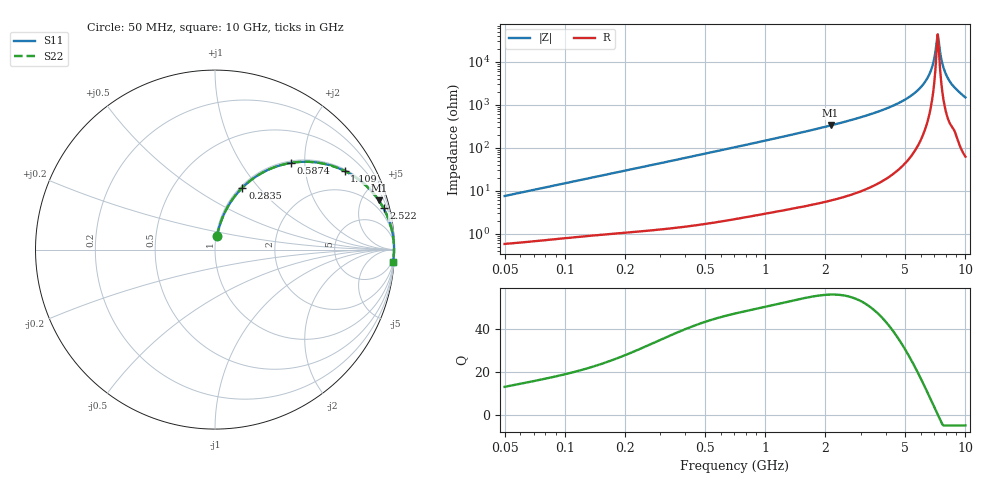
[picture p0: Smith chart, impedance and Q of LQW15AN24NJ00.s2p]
!Murata Part Number: LQW15AN24NJ00
!These Parameters are Measured in Series Mode Connection
!  o--[Z]--o
!Port1  Port2
!  o-------o
!Freq. Start=50[MHz] Stop=10[GHz], 401[Steps]
# Hz S RI R 50
!Freq.(Hz)	S 11(Real)	S 11(Imag)	S 21(Real)	S 21(Imag)	S 12(Real)	S 12(Imag)	S 22(Real)	S 22(Imag)
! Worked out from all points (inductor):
!   401 points, 50 MHz to 10 GHz, reference 50 ohm
!   read as one part in series: L = 23.7 nH near 51.34 MHz
!   highest Q = 56.1 at 2.123 GHz (marker M1), where L = 24.7 nH
!   self-resonance near 7.277 GHz
!   S11 on the Smith chart (normalised r, x): 50 MHz: 1.01, +0.15; 283.5 MHz: 1.02, +0.82; 587.4 MHz: 1.04, +1.71; 1.109 GHz: 1.06, +3.25; 2.522 GHz: 1.15, +8.13; 10 GHz: 2, -30
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5e7  0.0112 0.0737  0.9888 -0.0737  0.9888 -0.0737  0.0112 0.0737
1.214486e8  0.0387 0.1705  0.9613 -0.1705  0.9613 -0.1705  0.0387 0.1705
2.835028e8  0.1527 0.3453  0.8473 -0.3453  0.8473 -0.3453  0.1527 0.3453
2.949953e8  0.1626 0.3549  0.8374 -0.3549  0.8374 -0.3549  0.1626 0.3549
5.874203e8  0.423 0.4831  0.577 -0.4831  0.577 -0.4831  0.423 0.4831
7.071068e8  0.5136 0.4894  0.4864 -0.4894  0.4864 -0.4894  0.5136 0.4894
1.10936e9  0.7221 0.4383  0.2779 -0.4383  0.2779 -0.4383  0.7221 0.4383
1.717543e9  0.8661 0.3316  0.1339 -0.3316  0.1339 -0.3316  0.8661 0.3316
2.122994e9  0.9118 0.2748  0.0882 -0.2748  0.0882 -0.2748  0.9118 0.2748
2.521925e9  0.9393 0.2299  0.0607 -0.2299  0.0607 -0.2299  0.9393 0.2299
4.171863e9  0.9844 0.1123  0.0156 -0.1123  0.0156 -0.1123  0.9844 0.1123
5.225452e9  0.9932 0.0658  0.00676 -0.0658  0.00676 -0.0658  0.9932 0.0658
6.125686e9  0.9965 0.0342  0.00345 -0.0342  0.00345 -0.0342  0.9965 0.0342
6.720828e9  0.9975 0.0158  0.00251 -0.0158  0.00251 -0.0158  0.9975 0.0158
6.901252e9  0.9976 0.0106  0.00238 -0.0106  0.00238 -0.0106  0.9976 0.0106
7.086521e9  0.9977 0.00532  0.0023 -0.00532  0.0023 -0.00532  0.9977 0.00532
7.276762e9  0.9977 2.06e-05  0.0023 -2.06e-05  0.0023 -2.06e-05  0.9977 2.06e-05
7.472112e9  0.9976 -0.00531  0.00236 0.00531  0.00236 0.00531  0.9976 -0.00531
7.775012e9  0.9974 -0.0134  0.00262 0.0134  0.00262 0.0134  0.9974 -0.0134
8.198065e9  0.9966 -0.0243  0.00338 0.0243  0.00338 0.0243  0.9966 -0.0243
8.876195e9  0.9947 -0.0399  0.00534 0.0399  0.00534 0.0399  0.9947 -0.0399
1e10  0.9927 -0.0665  0.00725 0.0665  0.00725 0.0665  0.9927 -0.0665
